(* Logix 5000 AddOnInstructionDefinition export GracoCore_DecodeDateTime; software revision 32.04; part 4 of 4 *)

ADD_ON_INSTRUCTION GracoPd2kDual_WriteRecipe   (* revision 1.0 *)
// Help:
// Configures the values for a recipe number.
// Values outside of acceptable ranges will result in an error being raised.
// For mixRatioSP, the value corresponds to the ratio antecedent, i.e. the material A amount. For example, a value of 2.5 corresponds to a ratio of 2.5:1 (material A to material B). For single component recipes, set the value to 0. The max precision is two decimal places; anything beyond that will be rounded off.
// State Codes:
// * 0000 (IDLE) - Idle
// * 1000 (BUSY) - Busy
// * 2000 (DONE) - Done
// * 4000 (ABORT) - Command overwritten by another process
// * 8000 (ERROR) - Invalid input ranges
// * 8001 (ERROR) - Timeout waiting for DCS registers
// * 8002 (ERROR) - Command unsuccessful
// * 8003 (ERROR) - Unhandled internal error
VAR_INPUT
   i_execute : BOOL; {visible}   // Execute command
   i_mixUnitNum : DINT; {visible}   // Mix unit number
   i_recipeNum : DINT; {visible}   // Recipe number
   i_materialA : DINT; {visible}   // Material A
   i_materialB : DINT; {visible}   // Material B
   i_flushSeqA : DINT; {visible}   // Flush sequence A
   i_flushSeqB : DINT; {visible}   // Flush sequence B
   i_mixRatioSP : REAL; {visible}   // Mix ratio setpoint (A:B)
   i_potLifeTimeSP : DINT; {visible}   // Pot life time setpoint (min)
   i_mixPressureTol : DINT; {visible}   // Mix pressure tolerance (%)
END_VAR
VAR_OUTPUT
   o_busy : BOOL; {access Read Only, visible}   // Busy flag
   o_done : BOOL; {access Read Only, visible}   // Done flag
   o_aborted : BOOL; {access Read Only, visible}   // Aborted flag
   o_error : BOOL; {access Read Only, visible}   // Error flag
   o_state : DINT; {access Read Only, visible}   // Command state
END_VAR
VAR_IN_OUT
   io_moduleStatus : DINT[62]; {required}   // Data from device to PLC
   io_moduleCmds : DINT[30]; {required}   // Data from PLC to device
END_VAR
VAR
   sendDCSInst : GracoPd2kDual_SendDCS; {access None}   // SendDCS instruction
END_VAR

ROUTINE Logic   (* ladder *)
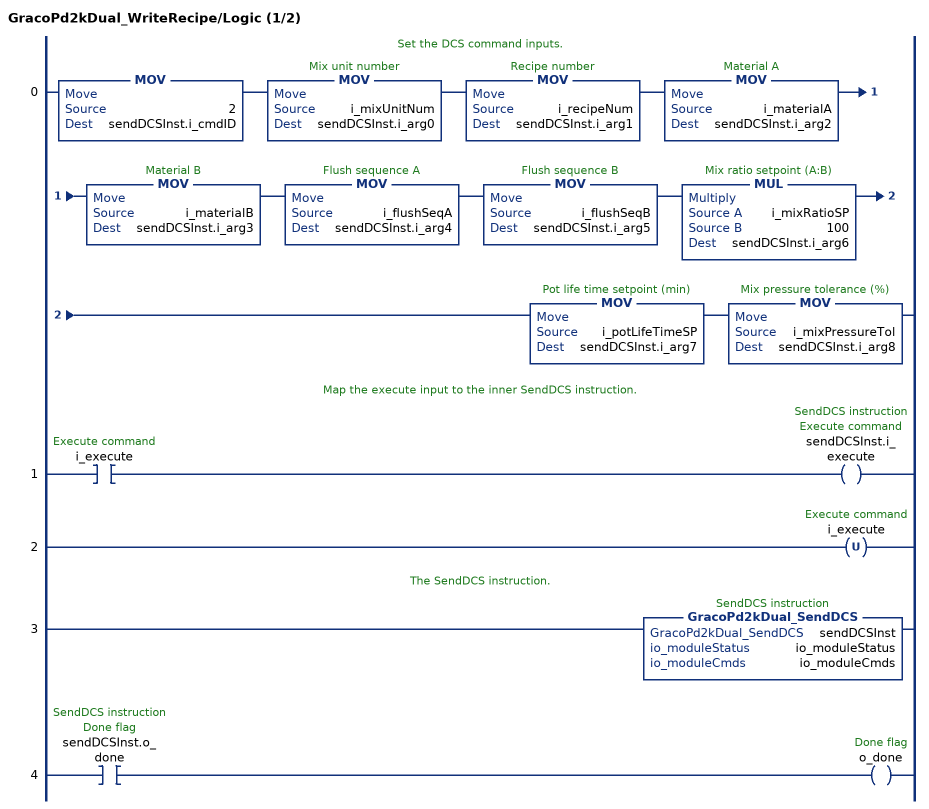
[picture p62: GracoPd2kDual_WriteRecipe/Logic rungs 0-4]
   // Set the DCS command inputs.
   0: MOV(2,sendDCSInst.i_cmdID)MOV(i_mixUnitNum,sendDCSInst.i_arg0)MOV(i_recipeNum,sendDCSInst.i_arg1)MOV(i_materialA,sendDCSInst.i_arg2)MOV(i_materialB,sendDCSInst.i_arg3)MOV(i_flushSeqA,sendDCSInst.i_arg4)MOV(i_flushSeqB,sendDCSInst.i_arg5)MUL(i_mixRatioSP,100,sendDCSInst.i_arg6)MOV(i_potLifeTimeSP,sendDCSInst.i_arg7)MOV(i_mixPressureTol,sendDCSInst.i_arg8);
   // Map the execute input to the inner SendDCS instruction.
   1: XIC(i_execute)OTE(sendDCSInst.i_execute);
   2: OTU(i_execute);
   // The SendDCS instruction.
   3: GracoPd2kDual_SendDCS(sendDCSInst,io_moduleStatus,io_moduleCmds);
   4: XIC(sendDCSInst.o_done)OTE(o_done);
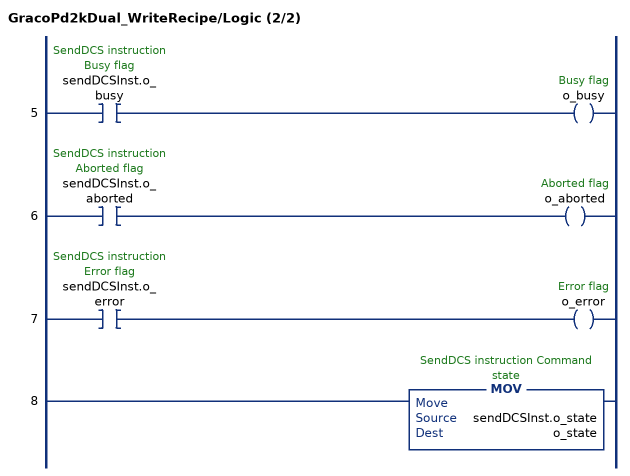
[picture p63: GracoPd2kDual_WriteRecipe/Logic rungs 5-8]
   5: XIC(sendDCSInst.o_busy)OTE(o_busy);
   6: XIC(sendDCSInst.o_aborted)OTE(o_aborted);
   7: XIC(sendDCSInst.o_error)OTE(o_error);
   8: MOV(sendDCSInst.o_state,o_state);
END_ROUTINE
END_ADD_ON_INSTRUCTION

ADD_ON_INSTRUCTION GracoPd2kDual_StatusToUDT   (* revision 1.0 *)
// Help:
// Returns structured data from the module as a UDT.
VAR_IN_OUT
   io_moduleStatus : DINT[62]; {required}   // Data from device to PLC
   io_statusUDT : GracoPd2kDual_TypePd2kDualStatus; {required}   // Status UDT
END_VAR

ROUTINE Logic   (* ladder *)
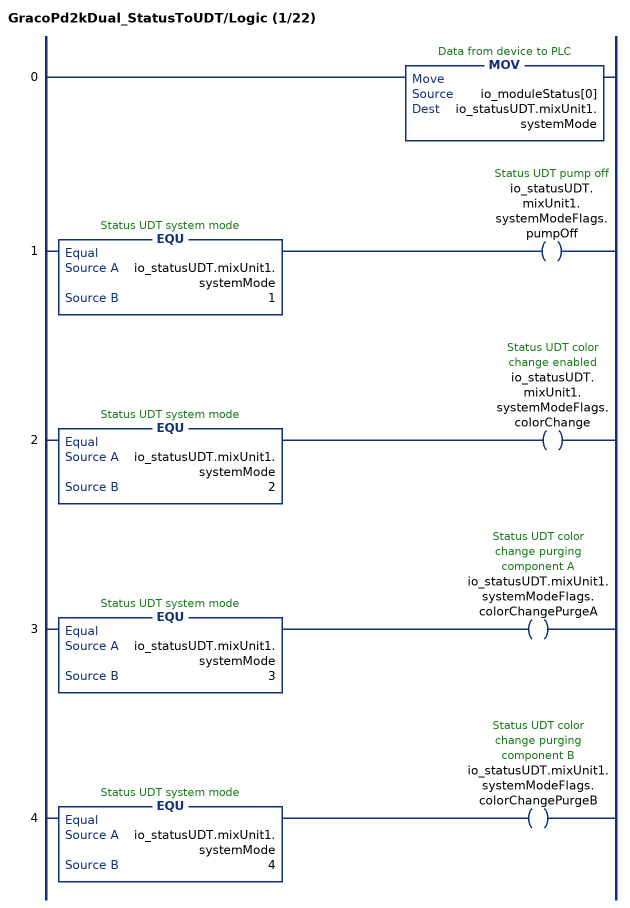
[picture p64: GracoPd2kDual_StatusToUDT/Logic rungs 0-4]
   0: MOV(io_moduleStatus[0],io_statusUDT.mixUnit1.systemMode);
   1: EQU(io_statusUDT.mixUnit1.systemMode,1)OTE(io_statusUDT.mixUnit1.systemModeFlags.pumpOff);
   2: EQU(io_statusUDT.mixUnit1.systemMode,2)OTE(io_statusUDT.mixUnit1.systemModeFlags.colorChange);
   3: EQU(io_statusUDT.mixUnit1.systemMode,3)OTE(io_statusUDT.mixUnit1.systemModeFlags.colorChangePurgeA);
   4: EQU(io_statusUDT.mixUnit1.systemMode,4)OTE(io_statusUDT.mixUnit1.systemModeFlags.colorChangePurgeB);
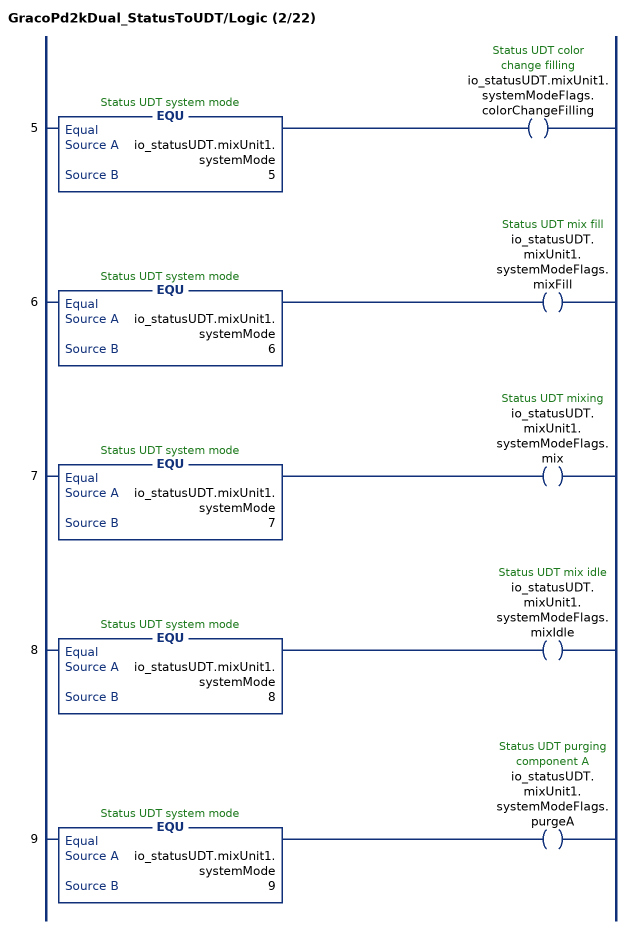
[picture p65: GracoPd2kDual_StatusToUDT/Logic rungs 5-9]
   5: EQU(io_statusUDT.mixUnit1.systemMode,5)OTE(io_statusUDT.mixUnit1.systemModeFlags.colorChangeFilling);
   6: EQU(io_statusUDT.mixUnit1.systemMode,6)OTE(io_statusUDT.mixUnit1.systemModeFlags.mixFill);
   7: EQU(io_statusUDT.mixUnit1.systemMode,7)OTE(io_statusUDT.mixUnit1.systemModeFlags.mix);
   8: EQU(io_statusUDT.mixUnit1.systemMode,8)OTE(io_statusUDT.mixUnit1.systemModeFlags.mixIdle);
   9: EQU(io_statusUDT.mixUnit1.systemMode,9)OTE(io_statusUDT.mixUnit1.systemModeFlags.purgeA);
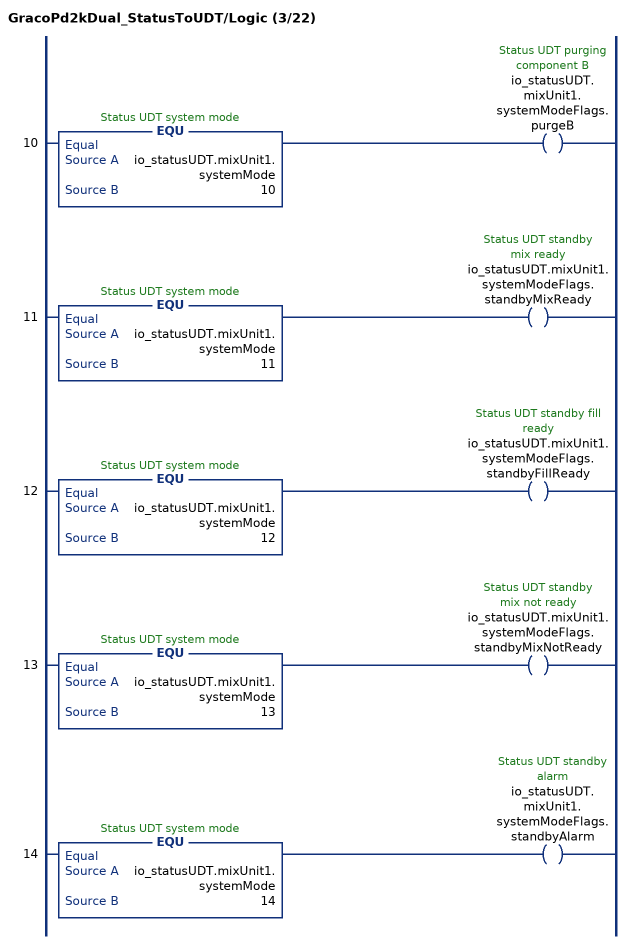
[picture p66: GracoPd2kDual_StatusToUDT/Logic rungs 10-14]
   10: EQU(io_statusUDT.mixUnit1.systemMode,10)OTE(io_statusUDT.mixUnit1.systemModeFlags.purgeB);
   11: EQU(io_statusUDT.mixUnit1.systemMode,11)OTE(io_statusUDT.mixUnit1.systemModeFlags.standbyMixReady);
   12: EQU(io_statusUDT.mixUnit1.systemMode,12)OTE(io_statusUDT.mixUnit1.systemModeFlags.standbyFillReady);
   13: EQU(io_statusUDT.mixUnit1.systemMode,13)OTE(io_statusUDT.mixUnit1.systemModeFlags.standbyMixNotReady);
   14: EQU(io_statusUDT.mixUnit1.systemMode,14)OTE(io_statusUDT.mixUnit1.systemModeFlags.standbyAlarm);
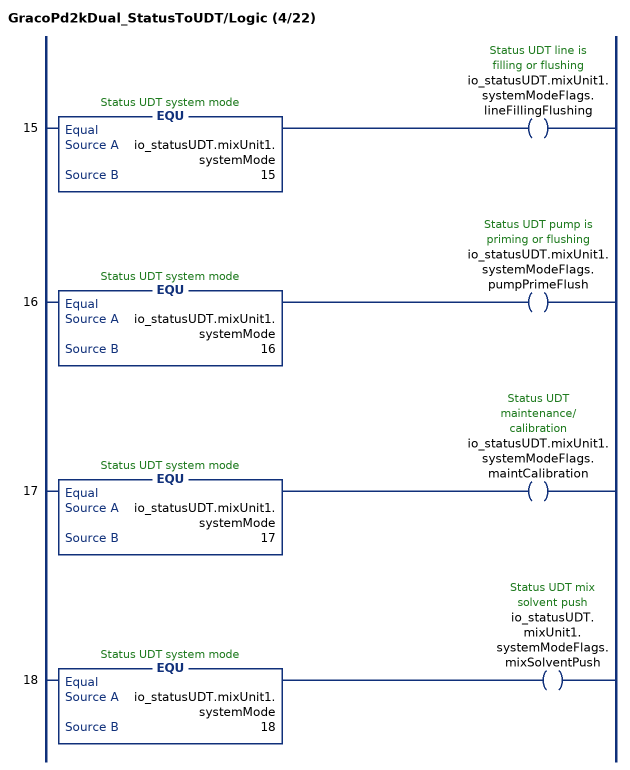
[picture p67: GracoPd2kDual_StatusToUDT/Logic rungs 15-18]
   15: EQU(io_statusUDT.mixUnit1.systemMode,15)OTE(io_statusUDT.mixUnit1.systemModeFlags.lineFillingFlushing);
   16: EQU(io_statusUDT.mixUnit1.systemMode,16)OTE(io_statusUDT.mixUnit1.systemModeFlags.pumpPrimeFlush);
   17: EQU(io_statusUDT.mixUnit1.systemMode,17)OTE(io_statusUDT.mixUnit1.systemModeFlags.maintCalibration);
   18: EQU(io_statusUDT.mixUnit1.systemMode,18)OTE(io_statusUDT.mixUnit1.systemModeFlags.mixSolventPush);
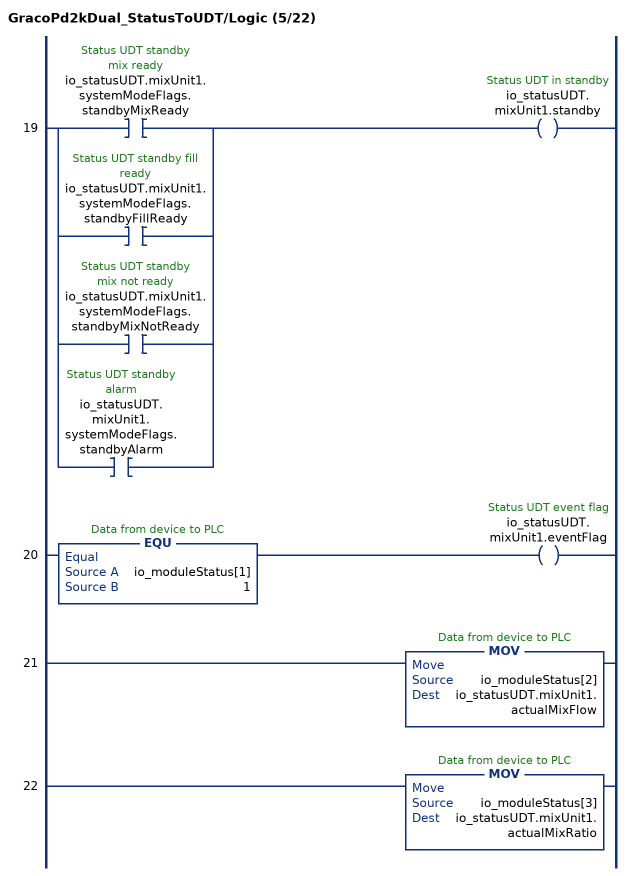
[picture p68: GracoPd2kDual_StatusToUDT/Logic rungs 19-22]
   19: [XIC(io_statusUDT.mixUnit1.systemModeFlags.standbyMixReady) ,XIC(io_statusUDT.mixUnit1.systemModeFlags.standbyFillReady) ,XIC(io_statusUDT.mixUnit1.systemModeFlags.standbyMixNotReady) ,XIC(io_statusUDT.mixUnit1.systemModeFlags.standbyAlarm) ]OTE(io_statusUDT.mixUnit1.standby);
   20: EQU(io_moduleStatus[1],1)OTE(io_statusUDT.mixUnit1.eventFlag);
   21: MOV(io_moduleStatus[2],io_statusUDT.mixUnit1.actualMixFlow);
   22: MOV(io_moduleStatus[3],io_statusUDT.mixUnit1.actualMixRatio);
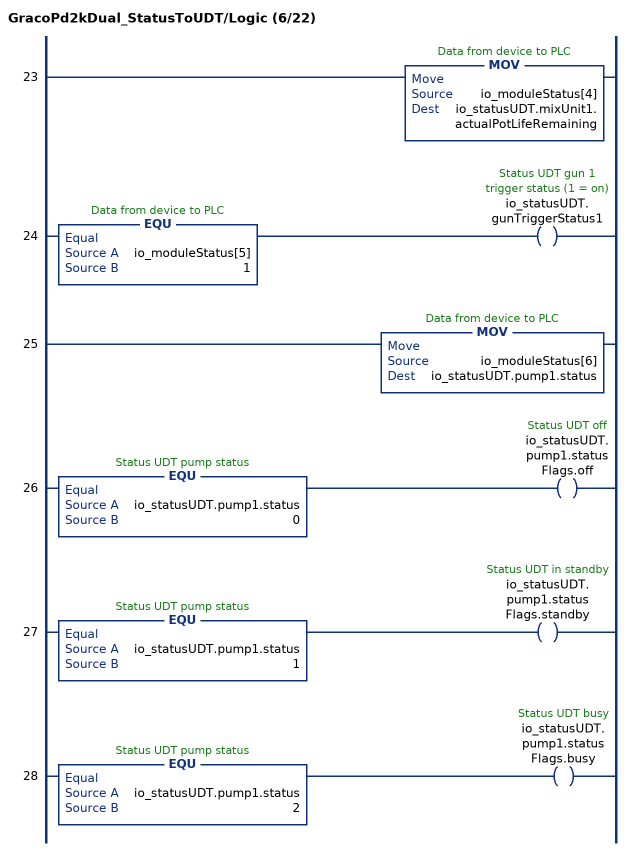
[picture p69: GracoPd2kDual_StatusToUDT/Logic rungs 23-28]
   23: MOV(io_moduleStatus[4],io_statusUDT.mixUnit1.actualPotLifeRemaining);
   24: EQU(io_moduleStatus[5],1)OTE(io_statusUDT.gunTriggerStatus1);
   25: MOV(io_moduleStatus[6],io_statusUDT.pump1.status);
   26: EQU(io_statusUDT.pump1.status,0)OTE(io_statusUDT.pump1.statusFlags.off);
   27: EQU(io_statusUDT.pump1.status,1)OTE(io_statusUDT.pump1.statusFlags.standby);
   28: EQU(io_statusUDT.pump1.status,2)OTE(io_statusUDT.pump1.statusFlags.busy);
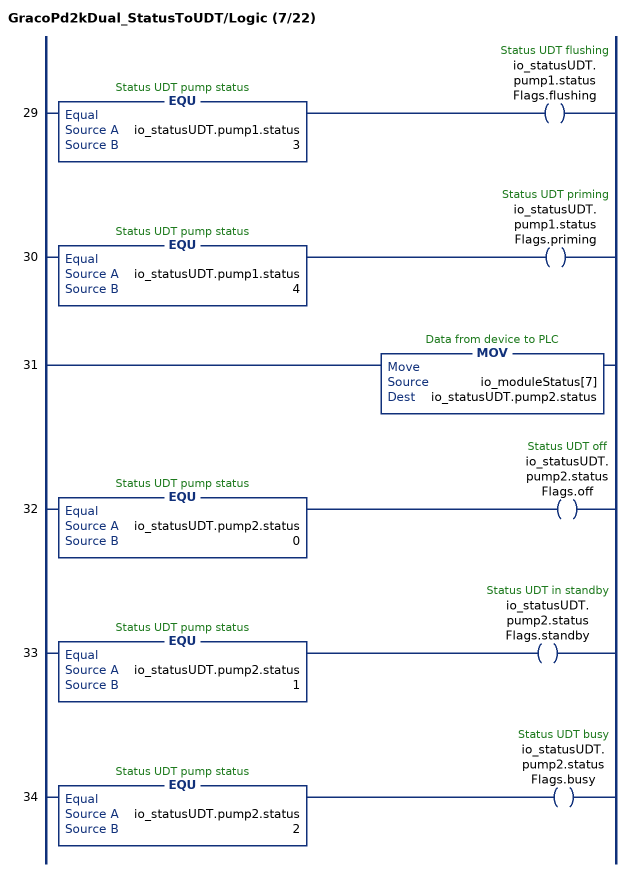
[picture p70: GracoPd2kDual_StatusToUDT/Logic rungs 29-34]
   29: EQU(io_statusUDT.pump1.status,3)OTE(io_statusUDT.pump1.statusFlags.flushing);
   30: EQU(io_statusUDT.pump1.status,4)OTE(io_statusUDT.pump1.statusFlags.priming);
   31: MOV(io_moduleStatus[7],io_statusUDT.pump2.status);
   32: EQU(io_statusUDT.pump2.status,0)OTE(io_statusUDT.pump2.statusFlags.off);
   33: EQU(io_statusUDT.pump2.status,1)OTE(io_statusUDT.pump2.statusFlags.standby);
   34: EQU(io_statusUDT.pump2.status,2)OTE(io_statusUDT.pump2.statusFlags.busy);
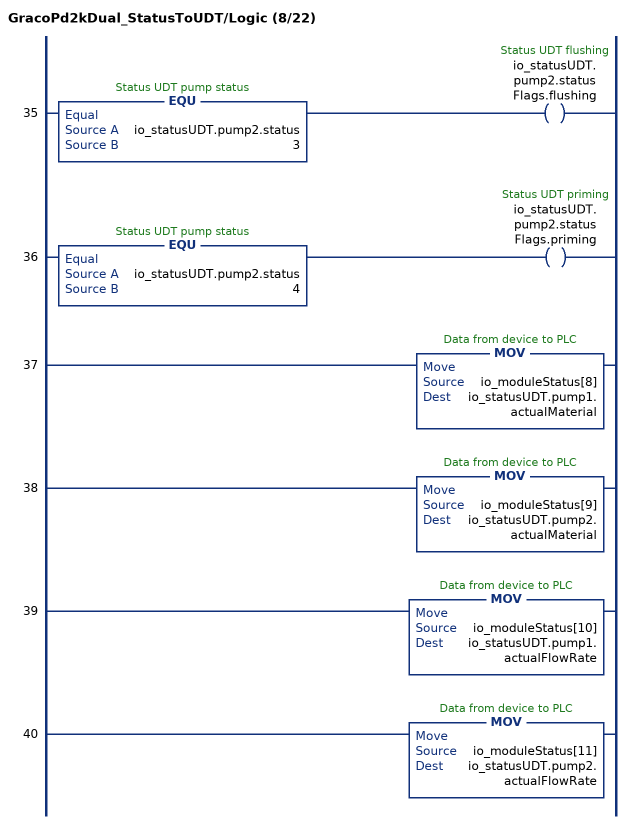
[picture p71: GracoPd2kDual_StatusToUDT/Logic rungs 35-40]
   35: EQU(io_statusUDT.pump2.status,3)OTE(io_statusUDT.pump2.statusFlags.flushing);
   36: EQU(io_statusUDT.pump2.status,4)OTE(io_statusUDT.pump2.statusFlags.priming);
   37: MOV(io_moduleStatus[8],io_statusUDT.pump1.actualMaterial);
   38: MOV(io_moduleStatus[9],io_statusUDT.pump2.actualMaterial);
   39: MOV(io_moduleStatus[10],io_statusUDT.pump1.actualFlowRate);
   40: MOV(io_moduleStatus[11],io_statusUDT.pump2.actualFlowRate);
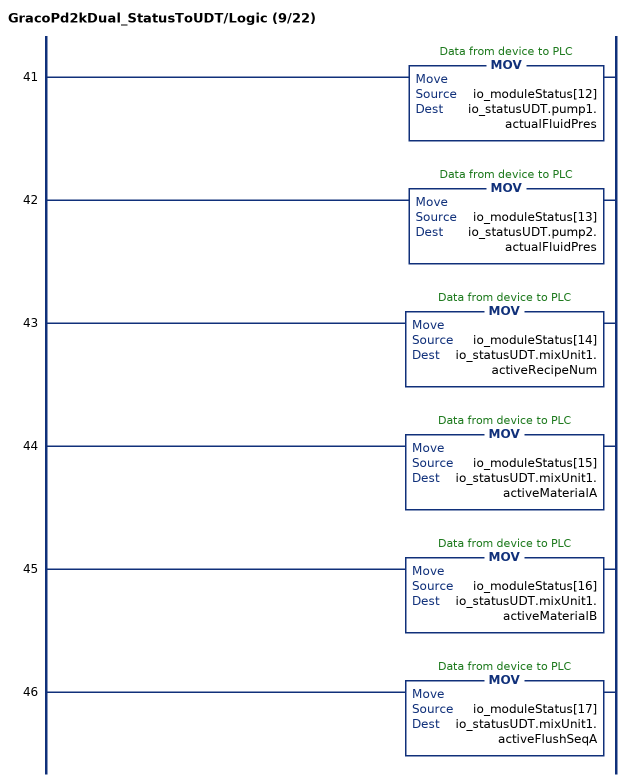
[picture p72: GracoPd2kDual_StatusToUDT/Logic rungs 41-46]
   41: MOV(io_moduleStatus[12],io_statusUDT.pump1.actualFluidPres);
   42: MOV(io_moduleStatus[13],io_statusUDT.pump2.actualFluidPres);
   43: MOV(io_moduleStatus[14],io_statusUDT.mixUnit1.activeRecipeNum);
   44: MOV(io_moduleStatus[15],io_statusUDT.mixUnit1.activeMaterialA);
   45: MOV(io_moduleStatus[16],io_statusUDT.mixUnit1.activeMaterialB);
   46: MOV(io_moduleStatus[17],io_statusUDT.mixUnit1.activeFlushSeqA);
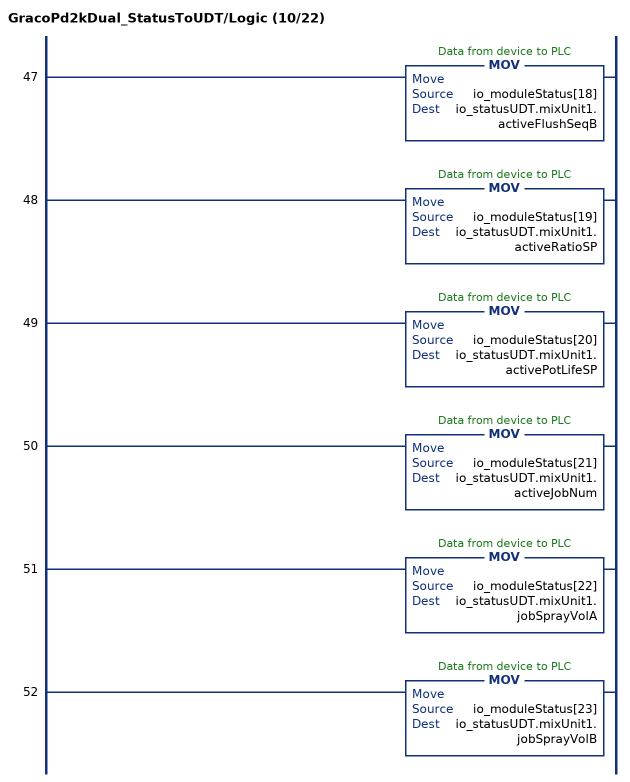
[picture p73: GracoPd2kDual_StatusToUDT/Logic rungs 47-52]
   47: MOV(io_moduleStatus[18],io_statusUDT.mixUnit1.activeFlushSeqB);
   48: MOV(io_moduleStatus[19],io_statusUDT.mixUnit1.activeRatioSP);
   49: MOV(io_moduleStatus[20],io_statusUDT.mixUnit1.activePotLifeSP);
   50: MOV(io_moduleStatus[21],io_statusUDT.mixUnit1.activeJobNum);
   51: MOV(io_moduleStatus[22],io_statusUDT.mixUnit1.jobSprayVolA);
   52: MOV(io_moduleStatus[23],io_statusUDT.mixUnit1.jobSprayVolB);
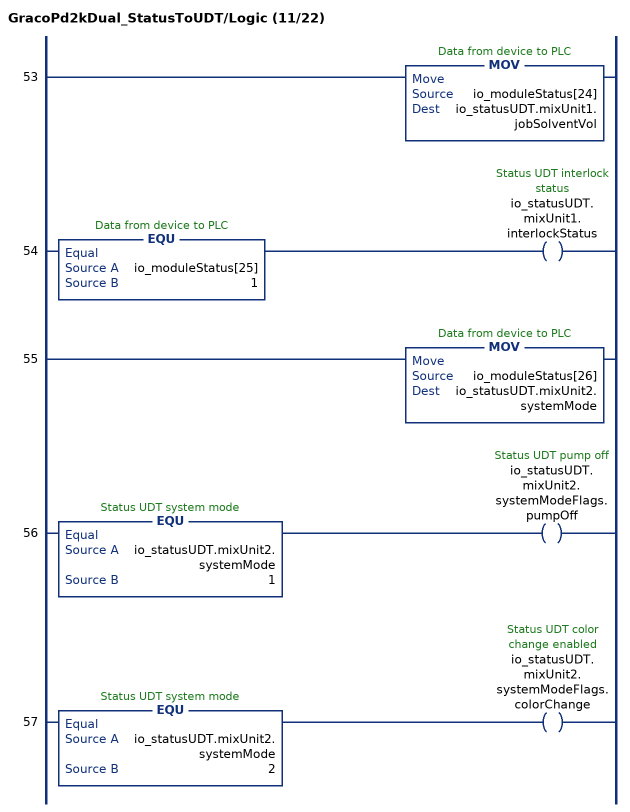
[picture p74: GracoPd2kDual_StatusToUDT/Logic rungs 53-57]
   53: MOV(io_moduleStatus[24],io_statusUDT.mixUnit1.jobSolventVol);
   54: EQU(io_moduleStatus[25],1)OTE(io_statusUDT.mixUnit1.interlockStatus);
   55: MOV(io_moduleStatus[26],io_statusUDT.mixUnit2.systemMode);
   56: EQU(io_statusUDT.mixUnit2.systemMode,1)OTE(io_statusUDT.mixUnit2.systemModeFlags.pumpOff);
   57: EQU(io_statusUDT.mixUnit2.systemMode,2)OTE(io_statusUDT.mixUnit2.systemModeFlags.colorChange);
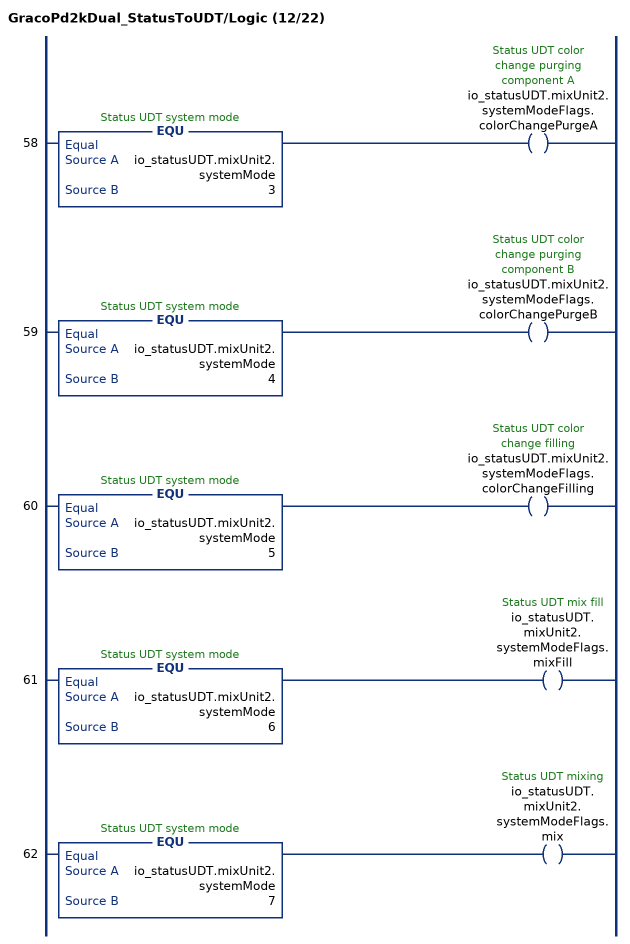
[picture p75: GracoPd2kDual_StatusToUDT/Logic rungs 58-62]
   58: EQU(io_statusUDT.mixUnit2.systemMode,3)OTE(io_statusUDT.mixUnit2.systemModeFlags.colorChangePurgeA);
   59: EQU(io_statusUDT.mixUnit2.systemMode,4)OTE(io_statusUDT.mixUnit2.systemModeFlags.colorChangePurgeB);
   60: EQU(io_statusUDT.mixUnit2.systemMode,5)OTE(io_statusUDT.mixUnit2.systemModeFlags.colorChangeFilling);
   61: EQU(io_statusUDT.mixUnit2.systemMode,6)OTE(io_statusUDT.mixUnit2.systemModeFlags.mixFill);
   62: EQU(io_statusUDT.mixUnit2.systemMode,7)OTE(io_statusUDT.mixUnit2.systemModeFlags.mix);
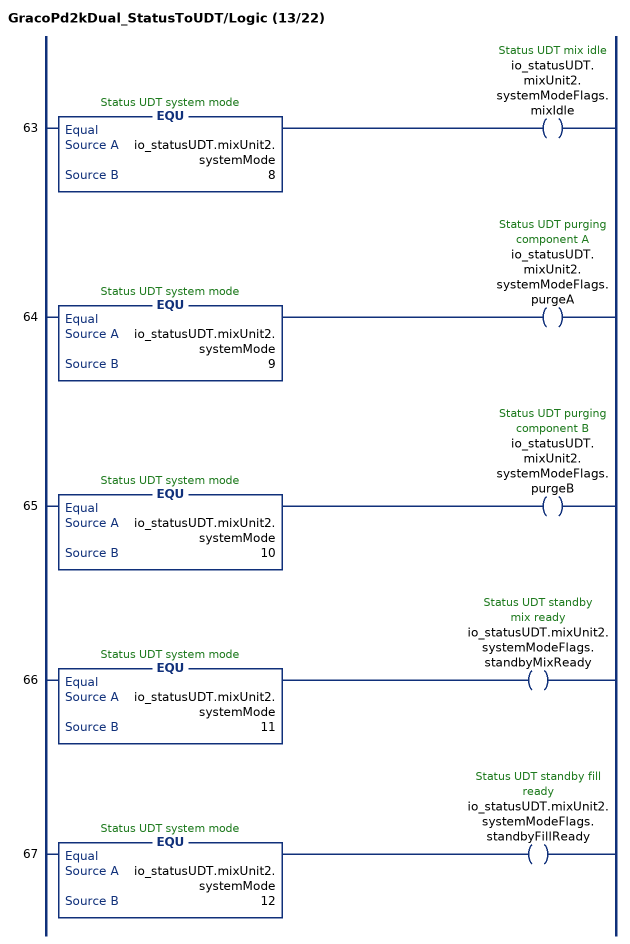
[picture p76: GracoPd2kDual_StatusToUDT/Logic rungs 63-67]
   63: EQU(io_statusUDT.mixUnit2.systemMode,8)OTE(io_statusUDT.mixUnit2.systemModeFlags.mixIdle);
   64: EQU(io_statusUDT.mixUnit2.systemMode,9)OTE(io_statusUDT.mixUnit2.systemModeFlags.purgeA);
   65: EQU(io_statusUDT.mixUnit2.systemMode,10)OTE(io_statusUDT.mixUnit2.systemModeFlags.purgeB);
   66: EQU(io_statusUDT.mixUnit2.systemMode,11)OTE(io_statusUDT.mixUnit2.systemModeFlags.standbyMixReady);
   67: EQU(io_statusUDT.mixUnit2.systemMode,12)OTE(io_statusUDT.mixUnit2.systemModeFlags.standbyFillReady);
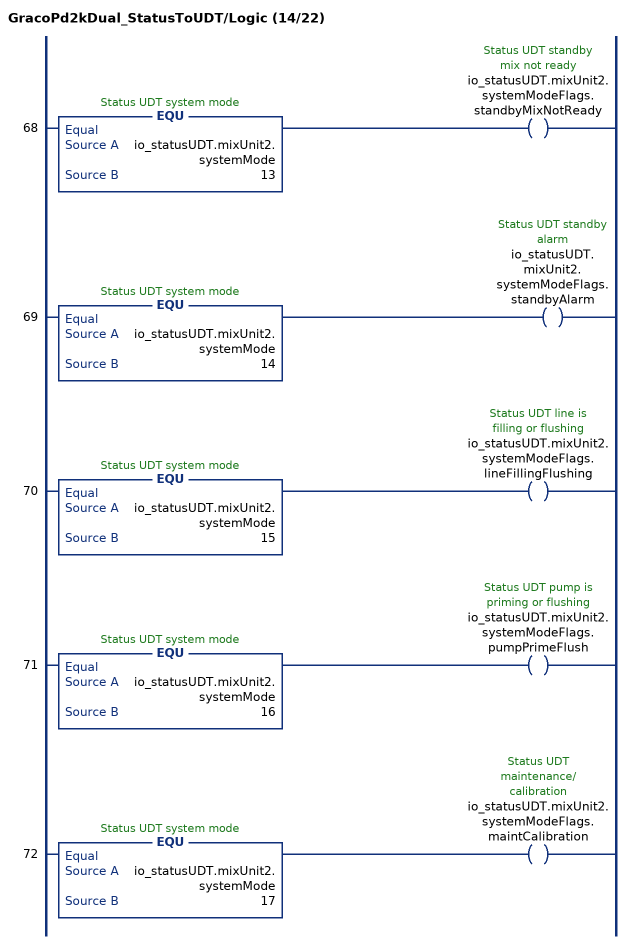
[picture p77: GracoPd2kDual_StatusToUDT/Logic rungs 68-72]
   68: EQU(io_statusUDT.mixUnit2.systemMode,13)OTE(io_statusUDT.mixUnit2.systemModeFlags.standbyMixNotReady);
   69: EQU(io_statusUDT.mixUnit2.systemMode,14)OTE(io_statusUDT.mixUnit2.systemModeFlags.standbyAlarm);
   70: EQU(io_statusUDT.mixUnit2.systemMode,15)OTE(io_statusUDT.mixUnit2.systemModeFlags.lineFillingFlushing);
   71: EQU(io_statusUDT.mixUnit2.systemMode,16)OTE(io_statusUDT.mixUnit2.systemModeFlags.pumpPrimeFlush);
   72: EQU(io_statusUDT.mixUnit2.systemMode,17)OTE(io_statusUDT.mixUnit2.systemModeFlags.maintCalibration);
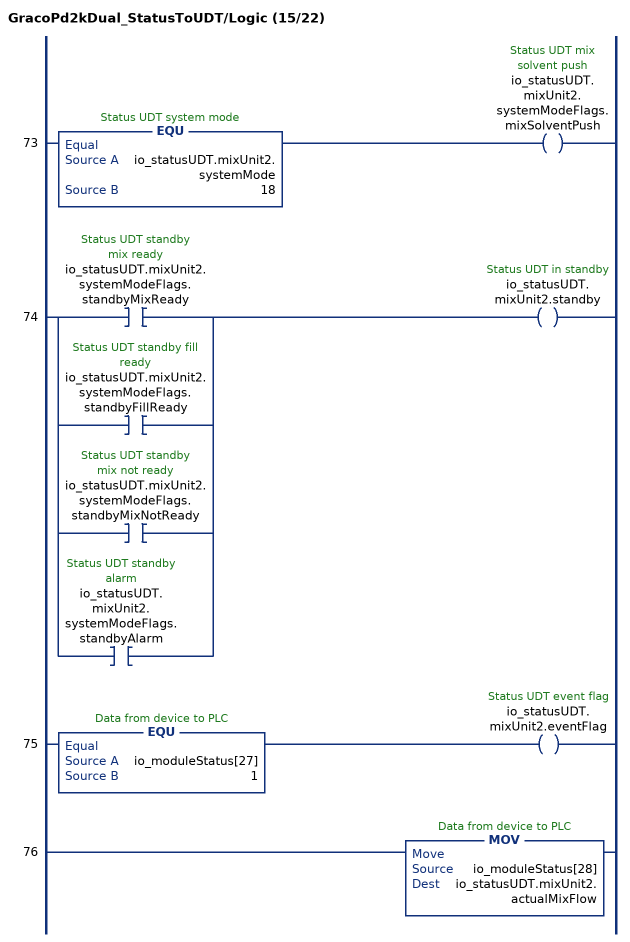
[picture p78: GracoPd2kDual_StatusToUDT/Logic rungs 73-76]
   73: EQU(io_statusUDT.mixUnit2.systemMode,18)OTE(io_statusUDT.mixUnit2.systemModeFlags.mixSolventPush);
   74: [XIC(io_statusUDT.mixUnit2.systemModeFlags.standbyMixReady) ,XIC(io_statusUDT.mixUnit2.systemModeFlags.standbyFillReady) ,XIC(io_statusUDT.mixUnit2.systemModeFlags.standbyMixNotReady) ,XIC(io_statusUDT.mixUnit2.systemModeFlags.standbyAlarm) ]OTE(io_statusUDT.mixUnit2.standby);
   75: EQU(io_moduleStatus[27],1)OTE(io_statusUDT.mixUnit2.eventFlag);
   76: MOV(io_moduleStatus[28],io_statusUDT.mixUnit2.actualMixFlow);
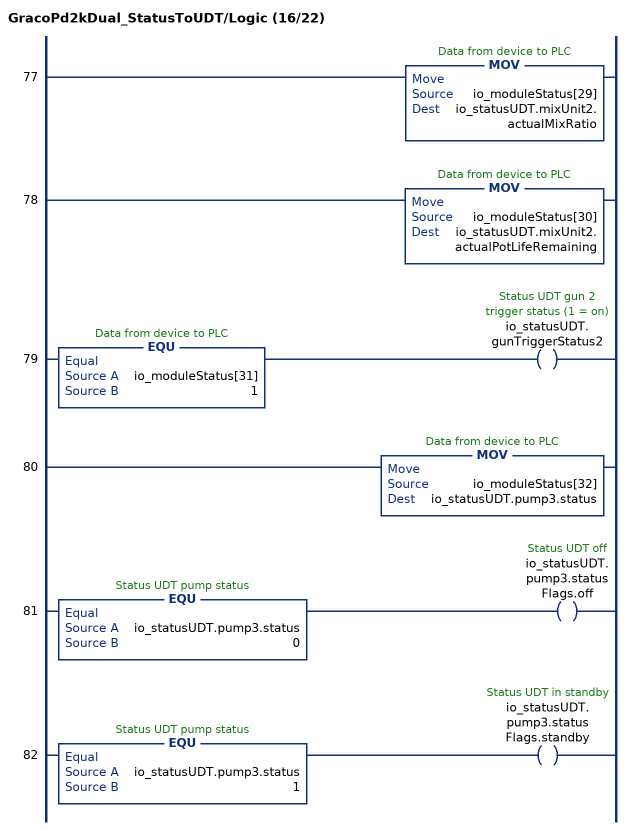
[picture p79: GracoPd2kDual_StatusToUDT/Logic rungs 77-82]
   77: MOV(io_moduleStatus[29],io_statusUDT.mixUnit2.actualMixRatio);
   78: MOV(io_moduleStatus[30],io_statusUDT.mixUnit2.actualPotLifeRemaining);
   79: EQU(io_moduleStatus[31],1)OTE(io_statusUDT.gunTriggerStatus2);
   80: MOV(io_moduleStatus[32],io_statusUDT.pump3.status);
   81: EQU(io_statusUDT.pump3.status,0)OTE(io_statusUDT.pump3.statusFlags.off);
   82: EQU(io_statusUDT.pump3.status,1)OTE(io_statusUDT.pump3.statusFlags.standby);
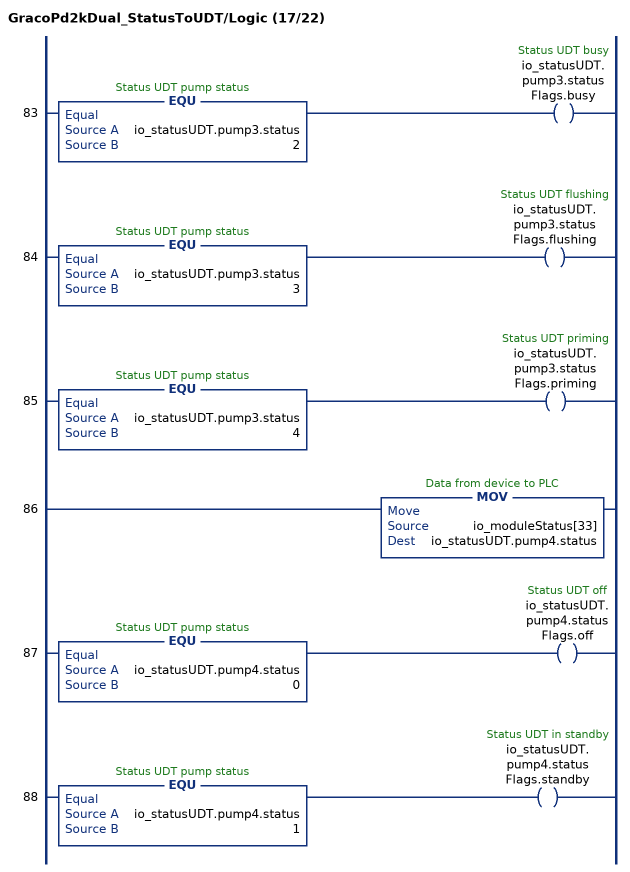
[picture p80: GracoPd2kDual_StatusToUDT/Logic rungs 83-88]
   83: EQU(io_statusUDT.pump3.status,2)OTE(io_statusUDT.pump3.statusFlags.busy);
   84: EQU(io_statusUDT.pump3.status,3)OTE(io_statusUDT.pump3.statusFlags.flushing);
   85: EQU(io_statusUDT.pump3.status,4)OTE(io_statusUDT.pump3.statusFlags.priming);
   86: MOV(io_moduleStatus[33],io_statusUDT.pump4.status);
   87: EQU(io_statusUDT.pump4.status,0)OTE(io_statusUDT.pump4.statusFlags.off);
   88: EQU(io_statusUDT.pump4.status,1)OTE(io_statusUDT.pump4.statusFlags.standby);
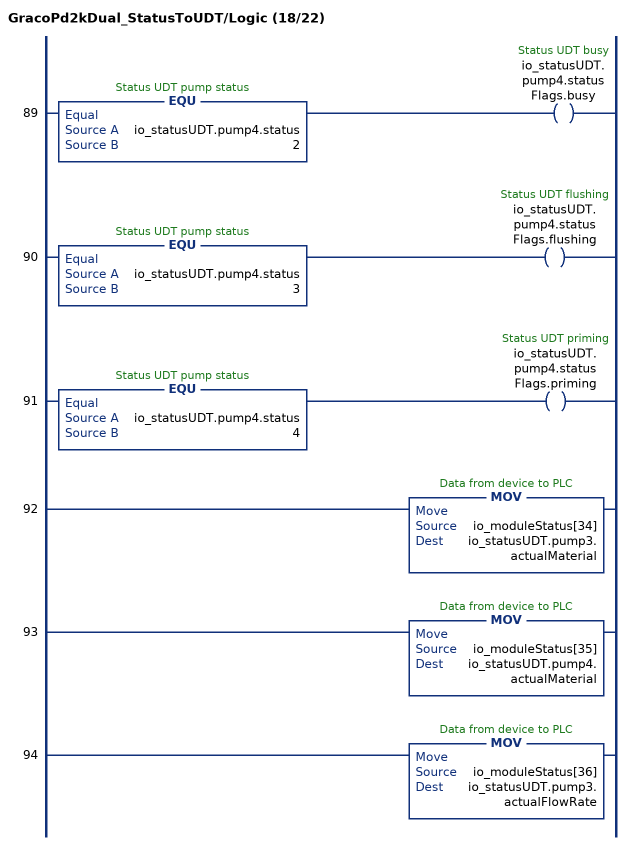
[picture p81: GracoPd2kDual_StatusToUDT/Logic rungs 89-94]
   89: EQU(io_statusUDT.pump4.status,2)OTE(io_statusUDT.pump4.statusFlags.busy);
   90: EQU(io_statusUDT.pump4.status,3)OTE(io_statusUDT.pump4.statusFlags.flushing);
   91: EQU(io_statusUDT.pump4.status,4)OTE(io_statusUDT.pump4.statusFlags.priming);
   92: MOV(io_moduleStatus[34],io_statusUDT.pump3.actualMaterial);
   93: MOV(io_moduleStatus[35],io_statusUDT.pump4.actualMaterial);
   94: MOV(io_moduleStatus[36],io_statusUDT.pump3.actualFlowRate);
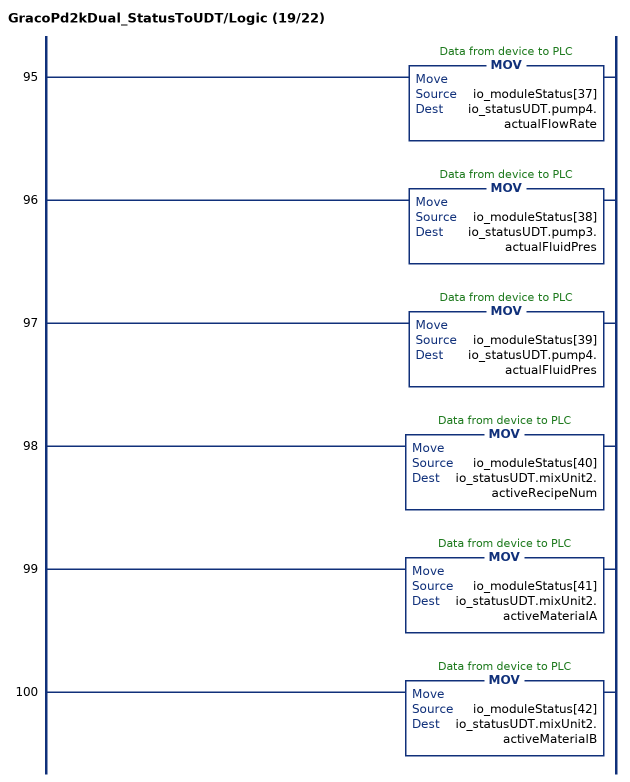
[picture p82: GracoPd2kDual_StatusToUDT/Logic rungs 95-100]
   95: MOV(io_moduleStatus[37],io_statusUDT.pump4.actualFlowRate);
   96: MOV(io_moduleStatus[38],io_statusUDT.pump3.actualFluidPres);
   97: MOV(io_moduleStatus[39],io_statusUDT.pump4.actualFluidPres);
   98: MOV(io_moduleStatus[40],io_statusUDT.mixUnit2.activeRecipeNum);
   99: MOV(io_moduleStatus[41],io_statusUDT.mixUnit2.activeMaterialA);
   100: MOV(io_moduleStatus[42],io_statusUDT.mixUnit2.activeMaterialB);
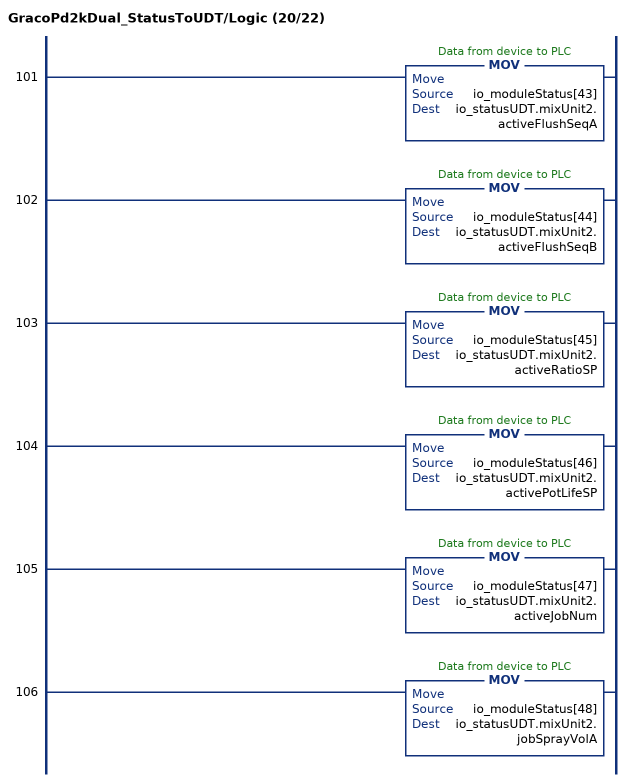
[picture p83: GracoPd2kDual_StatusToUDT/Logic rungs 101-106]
   101: MOV(io_moduleStatus[43],io_statusUDT.mixUnit2.activeFlushSeqA);
   102: MOV(io_moduleStatus[44],io_statusUDT.mixUnit2.activeFlushSeqB);
   103: MOV(io_moduleStatus[45],io_statusUDT.mixUnit2.activeRatioSP);
   104: MOV(io_moduleStatus[46],io_statusUDT.mixUnit2.activePotLifeSP);
   105: MOV(io_moduleStatus[47],io_statusUDT.mixUnit2.activeJobNum);
   106: MOV(io_moduleStatus[48],io_statusUDT.mixUnit2.jobSprayVolA);
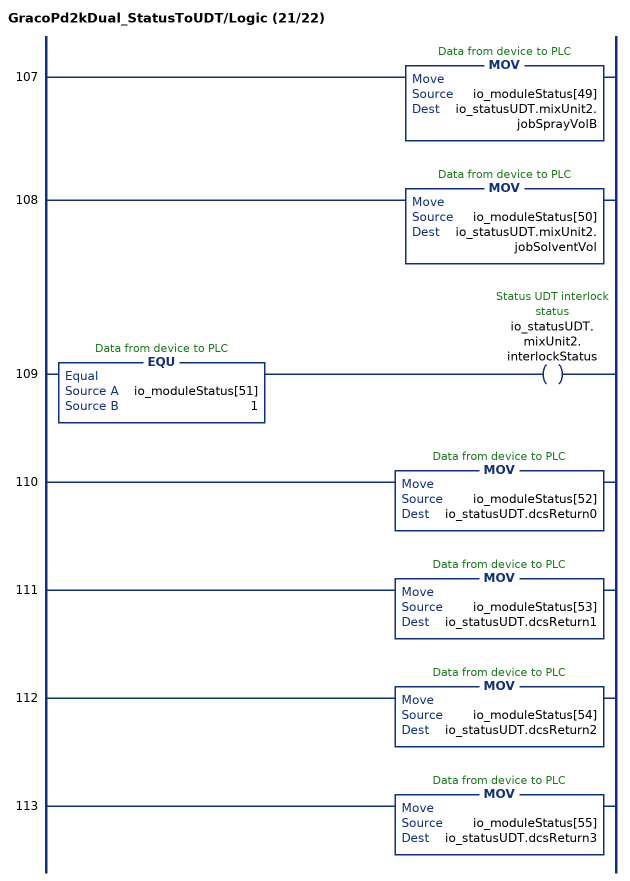
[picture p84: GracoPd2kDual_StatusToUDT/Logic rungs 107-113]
   107: MOV(io_moduleStatus[49],io_statusUDT.mixUnit2.jobSprayVolB);
   108: MOV(io_moduleStatus[50],io_statusUDT.mixUnit2.jobSolventVol);
   109: EQU(io_moduleStatus[51],1)OTE(io_statusUDT.mixUnit2.interlockStatus);
   110: MOV(io_moduleStatus[52],io_statusUDT.dcsReturn0);
   111: MOV(io_moduleStatus[53],io_statusUDT.dcsReturn1);
   112: MOV(io_moduleStatus[54],io_statusUDT.dcsReturn2);
   113: MOV(io_moduleStatus[55],io_statusUDT.dcsReturn3);
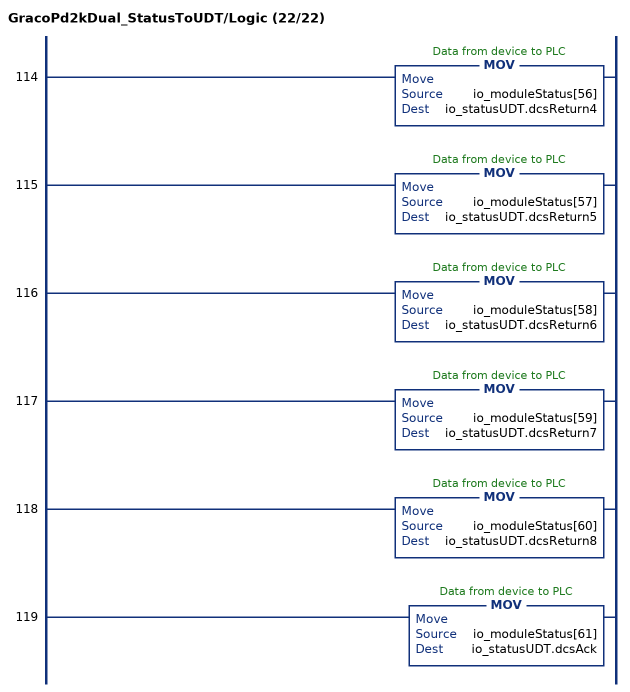
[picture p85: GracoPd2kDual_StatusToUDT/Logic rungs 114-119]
   114: MOV(io_moduleStatus[56],io_statusUDT.dcsReturn4);
   115: MOV(io_moduleStatus[57],io_statusUDT.dcsReturn5);
   116: MOV(io_moduleStatus[58],io_statusUDT.dcsReturn6);
   117: MOV(io_moduleStatus[59],io_statusUDT.dcsReturn7);
   118: MOV(io_moduleStatus[60],io_statusUDT.dcsReturn8);
   119: MOV(io_moduleStatus[61],io_statusUDT.dcsAck);
END_ROUTINE
END_ADD_ON_INSTRUCTION
